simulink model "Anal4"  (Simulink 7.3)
settings: Solver=ode45  StartTime=0.0  StopTime=10.0  RelTol=1e-3
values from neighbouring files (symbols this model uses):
  d2r = 1/r2d    (= 0.0174532925199)    [run.m]
  Kl3 = INFO.KFI(:,1:7)    [run.m]
  Thr = [470000, 470000, 470000, 0.245e7, 0.245e7]'    [run.m]
undefined symbols (not defined in the file or in its folder): Ap, Bp, Cp, Cyb, Dp, Mass, Qbar, Sref, TVC

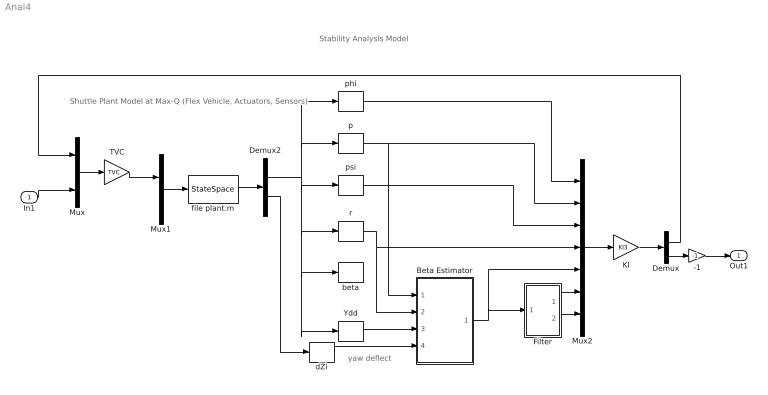
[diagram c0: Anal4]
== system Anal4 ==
  note: yaw deflect
  note: Shuttle Plant Model at Max-Q (Flex Vehicle, Actuators, Sensors)
  note: Stability Analysis Model
  In1 : Inport  OutDataType=sfix(16)  OutScaling=2^0
  -1 : Gain  Gain=-1  ParameterDataType=sfix(16)  ParameterScaling=2^0  OutDataType=sfix(16)  OutScaling=2^0
  Beta Estimator : Subsystem
  Demux : Demux  Outputs=2
  Demux2 : Demux  Outputs=[10, 20]
  Filter : Subsystem
  Kl : Gain  Gain=Kl3  Multiplication=Matrix(K*u)  ParameterDataType=sfix(16)  ParameterScaling=2^0  OutDataType=sfix(16)  OutScaling=2^0
  Mux : Mux  Inputs=3
  Mux1 : Mux  Inputs=[10,1]
  Mux2 : Mux  Inputs=7
  TVC : Gain  Gain=TVC  Multiplication=Matrix(K*u)  ParameterDataType=sfix(16)  ParameterScaling=2^0  OutDataType=sfix(16)  OutScaling=2^0
  Ydd : Selector  InputPortWidth=10  IndexOptions=Index vector (dialog)  Indices=[7]  OutputSizes=1
  beta : Selector  InputPortWidth=10  IndexOptions=Index vector (dialog)  Indices=[10]  OutputSizes=1
  dZi : Selector  InputPortWidth=20  IndexOptions=Index vector (dialog)  Indices=[16:20]  OutputSizes=1
  file plant.m : StateSpace  A=Ap  B=Bp  C=Cp  D=Dp
  p : Selector  InputPortWidth=10  IndexOptions=Index vector (dialog)  Indices=[4]  OutputSizes=1
  phi : Selector  InputPortWidth=10  IndexOptions=Index vector (dialog)  Indices=[1]  OutputSizes=1
  psi : Selector  InputPortWidth=10  IndexOptions=Index vector (dialog)  Indices=[3]  OutputSizes=1
  r : Selector  InputPortWidth=10  IndexOptions=Index vector (dialog)  Indices=[6]  OutputSizes=1
  Out1 : Outport  OutDataType=sfix(16)  OutScaling=2^0
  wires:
  Kl/1 -> Demux/1
  Mux2/1 -> Kl/1
  Filter/1(x1) -> Mux2/6
  Filter/2(x2) -> Mux2/7
  phi/1 -> Mux2/1
  p/1 -> Mux2/2, Beta Estimator/1(p)
  psi/1 -> Mux2/3
  r/1 -> Mux2/4, Beta Estimator/2(r)
  file plant.m/1 -> Demux2/1
  Demux2/1 -> r/1, beta/1, Ydd/1, psi/1, phi/1, p/1
  Mux1/1 -> file plant.m/1
  TVC/1 -> Mux1/1
  Mux/1 -> TVC/1
  Demux/1 -> Mux/1
  Demux2/2 -> dZi/1
  In1/1 -> Mux/3
  Demux/2 -> -1/1
  -1/1 -> Out1/1
  Beta Estimator/1(bethat) -> Mux2/5, Filter/1(bet)
  dZi/1 -> Beta Estimator/4(dz)
  Ydd/1 -> Beta Estimator/3(Ydd)

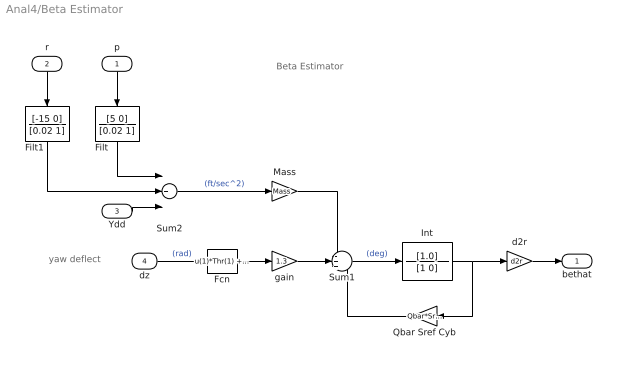
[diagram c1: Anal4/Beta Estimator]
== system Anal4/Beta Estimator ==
  note: yaw deflect
  note: Beta Estimator
  p : Inport
  r : Inport  Port=2
  Ydd : Inport  Port=3
  dz : Inport  Port=4  OutDataType=sfix(16)  OutScaling=2^0
  Fcn : Fcn  Expr=u(1)*Thr(1) +u(2)*Thr(2) +u(3)*Thr(3) +u(4)*Thr(4) +u(5)*Thr(5)
  Filt : TransferFcn  Numerator=[5 0]  Denominator=[0.02 1]
  Filt1 : TransferFcn  Numerator=[-15 0]  Denominator=[0.02 1]
  Int : TransferFcn  Numerator=[1.0]  Denominator=[1 0]
  Mass : Gain  Gain=Mass  ParameterDataType=sfix(16)  ParameterScaling=2^0  OutDataType=sfix(16)  OutScaling=2^0
  Qbar Sref Cyb : Gain  Gain=Qbar*Sref*Cyb  ParameterDataType=sfix(16)  ParameterScaling=2^0  OutDataType=sfix(16)  OutScaling=2^0
  Sum1 : Sum  Inputs=-++  OutDataType=sfix(16)  OutScaling=2^0
  Sum2 : Sum  Inputs=+++  OutDataType=sfix(16)  OutScaling=2^0
  d2r : Gain  Gain=d2r  ParameterDataType=sfix(16)  ParameterScaling=2^0  OutDataType=sfix(16)  OutScaling=2^0
  gain : Gain  Gain=1.3  ParameterDataType=sfix(16)  ParameterScaling=2^0  OutDataType=sfix(16)  OutScaling=2^0
  bethat : Outport  OutDataType=sfix(16)  OutScaling=2^0
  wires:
  p/1 -> Filt/1
  r/1 -> Filt1/1
  Ydd/1 -> Sum2/3
  gain/1 -> Sum1/2
  Fcn/1 -> gain/1
  Int/1 -> Qbar Sref Cyb/1, d2r/1
  d2r/1 -> bethat/1
  Mass/1 -> Sum1/1
  Sum2/1 -> Mass/1  "(ft/sec^2)"
  dz/1 -> Fcn/1  "(rad)"
  Qbar Sref Cyb/1 -> Sum1/3
  Sum1/1 -> Int/1  "(deg)"
  Filt1/1 -> Sum2/2
  Filt/1 -> Sum2/1

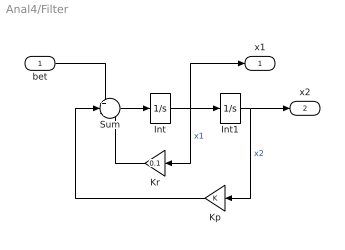
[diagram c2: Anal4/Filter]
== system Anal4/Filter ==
  bet : Inport  OutDataType=sfix(16)  OutScaling=2^0
  Int : Integrator
  Int1 : Integrator
  Kp : Gain  ParameterDataType=sfix(16)  ParameterScaling=2^0  OutDataType=sfix(16)  OutScaling=2^0
  Kr : Gain  Gain=0.1  ParameterDataType=sfix(16)  ParameterScaling=2^0  OutDataType=sfix(16)  OutScaling=2^0
  Sum : Sum  Inputs=+--  OutDataType=sfix(16)  OutScaling=2^0
  x1 : Outport  OutDataType=sfix(16)  OutScaling=2^0
  x2 : Outport  Port=2  OutDataType=sfix(16)  OutScaling=2^0
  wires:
  Int/1 -> Int1/1, Kr/1, x1/1  "x1"
  Sum/1 -> Int/1
  Int1/1 -> Kp/1, x2/1  "x2"
  Kr/1 -> Sum/3
  Kp/1 -> Sum/2
  bet/1 -> Sum/1
